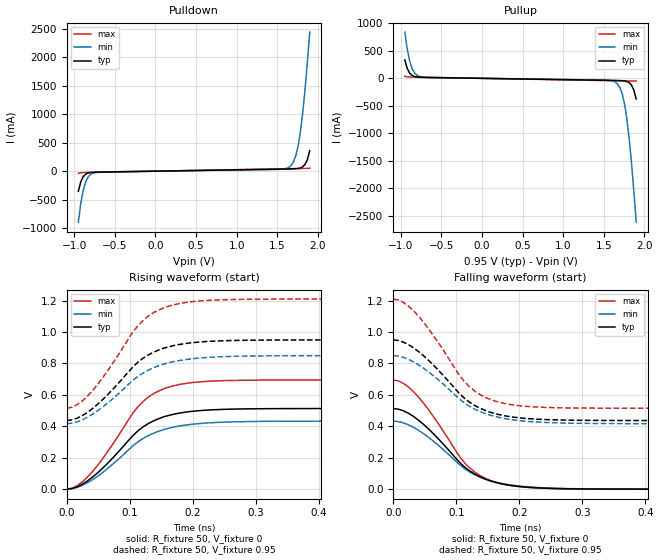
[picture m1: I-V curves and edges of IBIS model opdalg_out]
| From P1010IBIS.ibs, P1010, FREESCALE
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|The 004p has a 1.5x de-emphasis level.
|the 006p has a 2.0x de-emphasis level.
|PCI Express Gen 1 typically would use the 1.5x setting;
|PCI Express Gen 2 typically would use the 2.0x setting,
|but both are available on the device
[Model] opdalg_out
Model_type Output
Polarity Non-Inverting
Vref=0.95
Vmeas=0.475
C_comp   1.78pF   1.67pF   1.83pF
[Model Spec]
[Temperature Range] 65   125   -40
[Voltage Range]   0.95   0.85   1.21
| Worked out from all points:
|   slope of the pulldown table from 0 to 0.142 V, typ, clamps not added: 42.5 ohm
|   slope of the pullup table from 0 to 0.142 V, typ, clamps not added: 42.5 ohm
|   falling waveform, R_fixture 50, V_fixture 0: 20-80 % time 78.1ps typ, 82.2ps min, 74.1ps max; typ from 0.513 V to 0 V
|   falling waveform, R_fixture 50, V_fixture 0.95: 20-80 % time 78ps typ, 82.1ps min, 74.3ps max; typ from 0.95 V to 0.437 V
|   rising waveform, R_fixture 50, V_fixture 0: 20-80 % time 78.1ps typ, 82.2ps min, 74.3ps max; typ from 0 V to 0.513 V
|   rising waveform, R_fixture 50, V_fixture 0.95: 20-80 % time 78ps typ, 82.1ps min, 74ps max; typ from 0.437 V to 0.95 V
[Pullup]
-950mV    335.5mA    840.5mA    37.93mA
-920mV    177.7mA    532.3mA    28.21mA
-860mV    51.79mA    177.5mA    23.38mA
-810mV    26.34mA    67.84mA    21.83mA
-750mV    18.74mA    27.23mA    20.2mA
1.5V      -34.85mA   -31.69mA   -39.96mA
1.67V     -39.12mA   -102mA     -44.33mA
1.73V     -42.93mA   -293.4mA   -45.87mA
1.78V     -54.65mA   -682.7mA   -47.14mA
1.81V     -74.38mA   -1.045A    -47.9mA
1.84V     -117.8mA   -1.498A    -48.66mA
1.9V      -376.2mA   -2.614A    -50.18mA
[Pulldown]
-950mV    -354.6mA   -896.5mA   -37.95mA
-920mV    -186.1mA   -566.4mA   -28.15mA
-890mV    -96.12mA   -333.7mA   -24.84mA
-860mV    -52.71mA   -186.8mA   -23.38mA
-810mV    -26.35mA   -70.07mA   -21.83mA
-750mV    -18.71mA   -27.42mA   -20.2mA
1.5V      34.85mA    31.71mA    39.96mA
1.67V     39.13mA    98.9mA     44.33mA
1.73V     42.97mA    278.3mA    45.87mA
1.78V     54.49mA    642mA      47.14mA
1.84V     114.6mA    1.403A     48.66mA
1.9V      357.1mA    2.444A     50.18mA
[Falling Waveform]
R_fixture=50
V_fixture=0
V_fixture_min=0
V_fixture_max=0
0s        513.2mV    433.2mV    694.8mV
16.16ps   498.8mV    421.9mV    673.2mV
40.4ps    438.2mV    373.9mV    584.6mV
64.65ps   349.3mV    302.7mV    457.6mV
105.1ps   171.7mV    157.1mV    209.5mV
121.2ps   116.4mV    110.3mV    136mV
145.5ps   65.13mV    64.62mV    70.63mV
177.8ps   29.74mV    31.96mV    29.22mV
299ps     1.573mV    2.097mV    1.027mV
800ps     68.85nV    52.65nV    14.41nV
[Falling Waveform]
R_fixture=50
V_fixture=0.95
V_fixture_min=0.85
V_fixture_max=1.21
0s        950mV      850mV      1.21V
16.16ps   935.7mV    838.9mV    1.188V
40.4ps    875mV      790.8mV    1.1V
64.65ps   786.2mV    719.3mV    972.7mV
105.1ps   608.5mV    574mV      724.8mV
121.2ps   553.3mV    527.2mV    651.5mV
145.5ps   502mV      481.9mV    585.7mV
169.7ps   473.1mV    454.9mV    551.7mV
266.7ps   440.2mV    421.3mV    517.7mV
800ps     436.8mV    416.8mV    515.2mV
[Rising Waveform]
R_fixture=50
V_fixture=0
V_fixture_min=0
V_fixture_max=0
0s        6.854nV    32.41nV    1.012nV
16.16ps   14.42mV    11.17mV    21.48mV
40.4ps    75.21mV    59.24mV    110.4mV
64.65ps   164mV      130.8mV    237.4mV
105.1ps   341.5mV    276mV      485mV
121.2ps   396.9mV    322.8mV    558.5mV
145.5ps   448.1mV    368.2mV    623.8mV
177.8ps   483.4mV    401.1mV    665.5mV
290.9ps   511.4mV    430.6mV    693.5mV
800ps     513.2mV    433.2mV    694.8mV
[Rising Waveform]
R_fixture=50
V_fixture=0.95
V_fixture_min=0.85
V_fixture_max=1.21
0s        436.8mV    416.8mV    515.2mV
16.16ps   451.4mV    428.1mV    537.1mV
40.4ps    511.7mV    476mV      625.1mV
64.65ps   600.6mV    547.4mV    752.2mV
105.1ps   778.4mV    692.9mV    1.001V
121.2ps   833.8mV    739.5mV    1.074V
145.5ps   885mV      785.4mV    1.14V
177.8ps   920.4mV    818.1mV    1.181V
299ps     948.4mV    847.9mV    1.209V
800ps     950mV      850mV      1.21V
[Ramp]
R_load=50
dV/dt_r   3.079E-1/7.813E-11   2.599E-1/8.180E-11   4.169E-1/7.410E-11
dV/dt_f   3.079E-1/7.805E-11   2.599E-1/8.185E-11   4.169E-1/7.410E-11
| End [Model] opdalg_out
